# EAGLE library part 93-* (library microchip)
Serial EEPROM 512 x 8 bit/256 x 16 bit/1 K/4 K, 5.0 V, Microwire
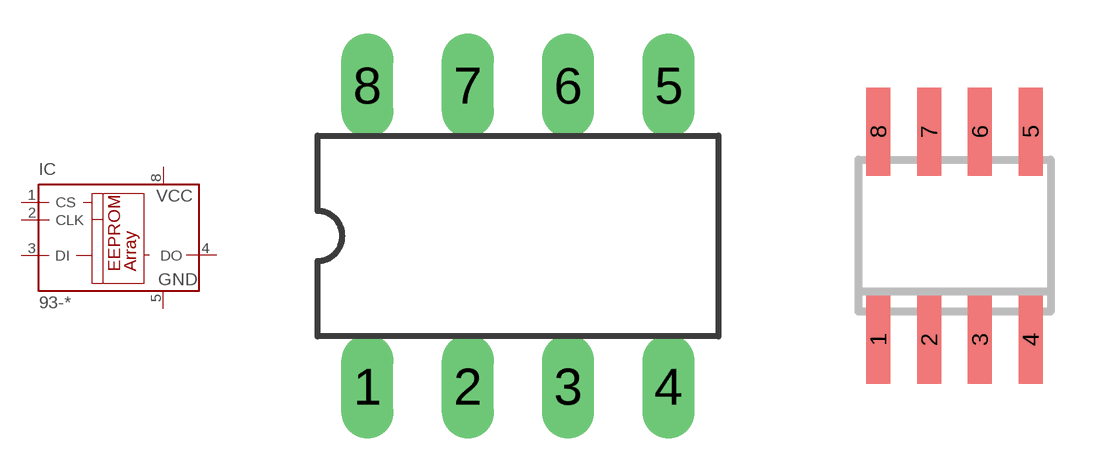
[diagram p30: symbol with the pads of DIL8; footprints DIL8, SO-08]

Designator prefix IC

## 93-C46AP (MF: MICROCHIP; MPN: 93C46A-I/P; OC_FARNELL: 1847808; OC_NEWARK: 92C7591), 93-C46BP (MF: MICROCHIP; MPN: 93C46B/P; OC_FARNELL: 1084337; OC_NEWARK: 69K7676), 93-C56AP (MF: MICROCHIP; MPN: 93C56A-E/P; OC_FARNELL: unknown; OC_NEWARK: 92C7619), 93-C56BP (MF: MICROCHIP; MPN: 93C56B-I/P; OC_FARNELL: 1718065; OC_NEWARK: 61H6567), 93-C66AP (MF: MICROCHIP; MPN: 93C66A-I/P; OC_FARNELL: 1818607; OC_NEWARK: 61H6596), 93-C66BP (MF: MICROCHIP; MPN: 93C66B-I/P; OC_FARNELL: 1818523; OC_NEWARK: 61H6625), 93-LC56AP (MF: MICROCHIP; MPN: 93LC56A/P; OC_FARNELL: 1212671; OC_NEWARK: 75K5894), 93-LC56BP (MF: MICROCHIP; MPN: 93LC56B/P; OC_FARNELL: 1084250; OC_NEWARK: 96K4108)  [DIL8]
1  CS  in
2  CLK  in
3  DI  in
4  DO  hiz
5  GND  pwr
8  VCC  pwr

## 93-C46ASN (MF: MICROCHIP; MPN: 93C46A-I/SN; OC_FARNELL: 1816075; OC_NEWARK: 92C7592), 93-C46BSN (MF: MICROCHIP; MPN: 93C46B/SN; OC_FARNELL: 9758178; OC_NEWARK: 75K5893), 93-C56ASN (MF: MICROCHIP; MPN: 93C56A-I/SN; OC_FARNELL: 1815962; OC_NEWARK: 61H6540), 93-C56BSN (MF: MICROCHIP; MPN: 93C56B-I/SN; OC_FARNELL: 1847100; OC_NEWARK: 61H6569), 93-C66ASN (MF: MICROCHIP; MPN: 93C66A-I/SN; OC_FARNELL: 1847311; OC_NEWARK: 61H6598), 93-C66BSN (OC_FARNELL: unknown; OC_NEWARK: unknown), 93-LC56ASN (MF: MICROCHIP; MPN: 93LC56A/SN; OC_FARNELL: 1212672; OC_NEWARK: 33C3019), 93-LC56BSN (MF: MICROCHIP; MPN: 93LC56B/SN; OC_FARNELL: 9758240; OC_NEWARK: 96K4109)  [SO-08]
Pads as for DIL8

## 93-C46AST (MPN: CAT93C46YI-G; OC_FARNELL: 1718375; OC_NEWARK: 74P0100), 93-C46BST (MF: MICROCHIP; MPN: 93C46B/ST; OC_FARNELL: unknown; OC_NEWARK: 92C7605), 93-LC56AST (MF: MICROCHIP; MPN: 93LC56A-E/ST; OC_FARNELL: unknown; OC_NEWARK: 30H4734), 93-LC56BST (MF: MICROCHIP; MPN: 93LC56B-E/ST; OC_FARNELL: unknown; OC_NEWARK: 30H4749)  [TSSOP8]
Pads as for DIL8

## 93-C46ASM (MF: MICROCHIP; MPN: 93C46A-I/SN; OC_FARNELL: 1816075; OC_NEWARK: 92C7592), 93-C46BSM (MF: MICROCHIP; MPN: 93C46B/SN; OC_FARNELL: 9758178; OC_NEWARK: 75K5893), 93-LC56ASM (MF: MICROCHIP; MPN: 93LC56A/SN; OC_FARNELL: 1212672; OC_NEWARK: 33C3019), 93-LC56BSM (MF: MICROCHIP; MPN: 93LC56B/SN; OC_FARNELL: 9758240; OC_NEWARK: 96K4109)  [SO-08M]
Pads as for DIL8

## Footprint DIL8 (pad centres in mm)
Dual In Line package type P
drill 0.813 long: 1 -3.81,-3.81; 2 -1.27,-3.81; 3 1.27,-3.81; 4 3.81,-3.81; 5 3.81,3.81; 6 1.27,3.81; 7 -1.27,3.81; 8 -3.81,3.81

## Footprint SO-08 (pad centres in mm)
Small Outline Narrow Plastic Gull Wing 150-mil body, package type SN
smd 0.6 x 2.2: 1 -1.905,-2.6; 2 -0.635,-2.6; 3 0.635,-2.6; 4 1.905,-2.6; 5 1.905,2.6; 6 0.635,2.6; 7 -0.635,2.6; 8 -1.905,2.6

## Footprint TSSOP8 (pad centres in mm)
Thin Shrink Small Outline Package package type ST
smd 0.35 x 1.2: 1 -0.975,-2.925; 2 -0.325,-2.925; 3 0.325,-2.925; 4 0.975,-2.925; 5 0.975,2.925; 6 0.325,2.925; 7 -0.325,2.925; 8 -0.975,2.925

## Footprint SO-08M (pad centres in mm)
Small Outline Medium Plastic Gull Wing 207-mil body, package type SM
smd 0.6 x 2.2: 1 -1.905,-3.33; 2 -0.635,-3.33; 3 0.635,-3.33; 4 1.905,-3.33; 5 1.905,3.33; 6 0.635,3.33; 7 -0.635,3.33; 8 -1.905,3.33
